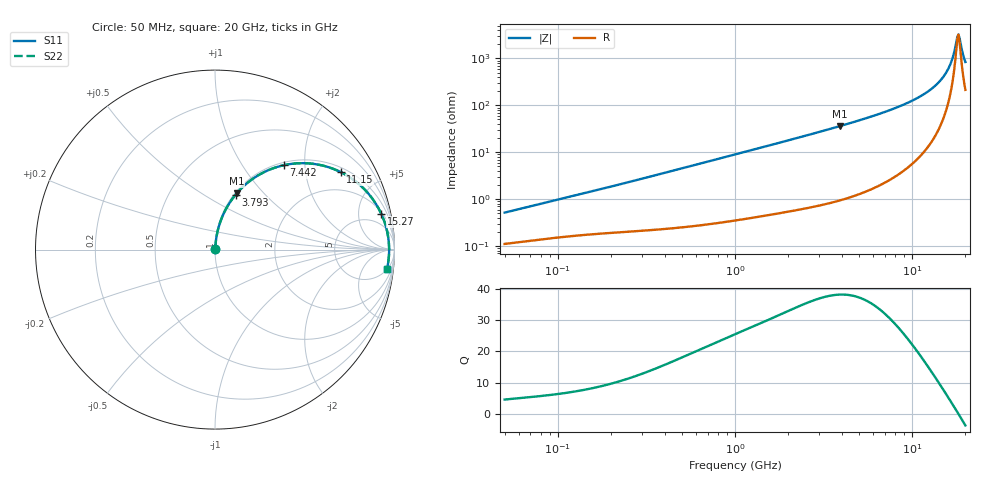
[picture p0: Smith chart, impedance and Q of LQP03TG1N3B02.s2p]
!Murata Part Number: LQP03TG1N3B02
!These Parameters are Measured in Series Mode Connection
!  o--[Z]--o
!Port1  Port2
!  o-------o
!Freq. Start=50[MHz] Stop=20[GHz], 401[Steps]
# Hz S RI R 50
!Freq.(Hz) S11(Real) S11(Imag) S21(Real) S21(Imag) S12(Real) S12(Imag) S22(Real) S22(Imag)
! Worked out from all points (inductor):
!   401 points, 50 MHz to 20 GHz, reference 50 ohm
!   read as one part in series: L = 1.58 nH near 51.52 MHz
!   highest Q = 38.3 at 3.908 GHz (marker M1), where L = 1.47 nH
!   self-resonance near 18.01 GHz
!   S11 on the Smith chart (normalised r, x): 50 MHz: 1.00, +0.01; 3.793 GHz: 1.02, +0.70; 7.442 GHz: 1.05, +1.57; 11.15 GHz: 1.17, +3.12; 15.27 GHz: 2.25, +8.80; 20 GHz: 5, -16
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5e7  0.00114 0.00505  0.9989 -0.00505  0.9989 -0.00505  0.00114 0.00505
1.364002e8  0.00188 0.0128  0.9981 -0.0128  0.9981 -0.0128  0.00188 0.0128
3.721004e8  0.0034 0.0337  0.9966 -0.0337  0.9966 -0.0337  0.0034 0.0337
1e9  0.0114 0.0884  0.9886 -0.0884  0.9886 -0.0884  0.0114 0.0884
2.728004e9  0.0629 0.2294  0.9371 -0.2294  0.9371 -0.2294  0.0629 0.2294
3.792786e9  0.115 0.3062  0.885 -0.3062  0.885 -0.3062  0.115 0.3062
3.908127e9  0.1215 0.3139  0.8785 -0.3139  0.8785 -0.3139  0.1215 0.3139
5.515528e9  0.228 0.406  0.772 -0.406  0.772 -0.406  0.228 0.406
7.442007e9  0.3845 0.4705  0.6155 -0.4705  0.6155 -0.4705  0.3845 0.4705
9.316812e9  0.5485 0.4777  0.4515 -0.4777  0.4515 -0.4777  0.5485 0.4777
1.115139e10  0.6996 0.4324  0.3004 -0.4324  0.3004 -0.4324  0.6996 0.4324
1.334722e10  0.8441 0.3239  0.1559 -0.3239  0.1559 -0.3239  0.8441 0.3239
1.438523e10  0.8938 0.2591  0.1062 -0.2591  0.1062 -0.2591  0.8938 0.2591
1.527346e10  0.9261 0.1999  0.0739 -0.1999  0.0739 -0.1999  0.9261 0.1999
1.597544e10  0.9451 0.152  0.0549 -0.152  0.0549 -0.152  0.9451 0.152
1.670968e10  0.959 0.1018  0.041 -0.1018  0.041 -0.1018  0.959 0.1018
1.774144e10  0.969 0.0324  0.031 -0.0324  0.031 -0.0324  0.969 0.0324
1.800918e10  0.9699 0.0149  0.0301 -0.0149  0.0301 -0.0149  0.9699 0.0149
1.828096e10  0.9702 -0.00274  0.0298 0.00274  0.0298 0.00274  0.9702 -0.00274
1.855685e10  0.9698 -0.0203  0.0302 0.0203  0.0302 0.0203  0.9698 -0.0203
1.940974e10  0.9649 -0.0728  0.0351 0.0728  0.0351 0.0728  0.9649 -0.0728
2e10  0.9585 -0.1073  0.0415 0.1073  0.0415 0.1073  0.9585 -0.1073
